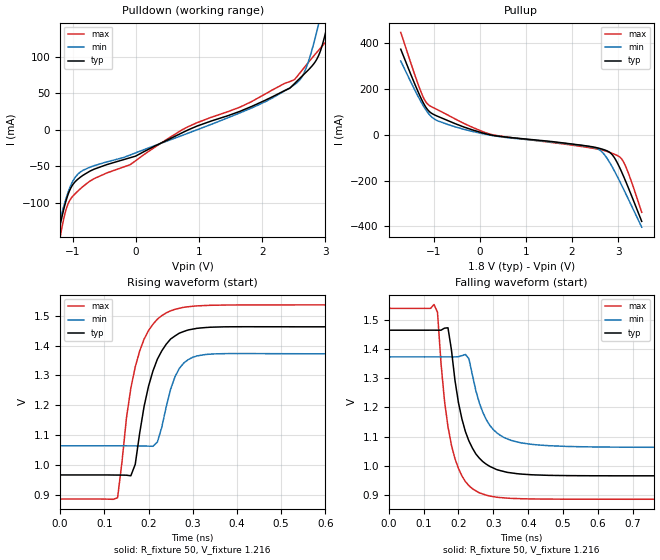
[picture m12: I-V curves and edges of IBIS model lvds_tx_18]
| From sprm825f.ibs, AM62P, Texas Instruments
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|   MODEL lvds_tx_18
[Model] lvds_tx_18
Model_type Output
C_comp 1.657p 1.754p 1.436p
Vmeas = 1.2
Vref = 1.2V
Rref = 50
Cref = 0.5pF
[Model Spec]
[Temperature Range]  40 150 -40
[Voltage Range] 1.8 1.62 1.98
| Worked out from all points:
|   slope of the pulldown table from 0 to 0.27 V, typ, clamps not added: 22.1 ohm
|   slope of the pullup table from 0 to 0.27 V, typ, clamps not added: 19.7 ohm
|   rising waveform, R_fixture 50, V_fixture 1.216: 20-80 % time 47.4ps typ, 35.3ps min, 46ps max; typ from 0.967 V to 1.46 V
|   falling waveform, R_fixture 50, V_fixture 1.216: 20-80 % time 54.9ps typ, 58.8ps min, 45.8ps max; typ from 1.46 V to 0.967 V
[Pulldown]
-1.71V    -377.9mA   -327mA     -450.5mA
-1.245V   -149.3mA   -138.7mA   -169.9mA
-1.193V   -127.2mA   -120.3mA   -143.1mA
-1.05V    -83.02mA   -79.84mA   -96.79mA
-838.9mV  -62.25mA   -55.44mA   -77.53mA
833.2mV   0A         -4.508mA   4.354mA
2.054V    40.45mA    38.4mA     49.03mA
2.624V    72.45mA    71.03mA    80.23mA
2.888V    99.94mA    141.8mA    107.9mA
3.03V     142mA      196.2mA    122.2mA
3.141V    189.6mA    241.3mA    140.8mA
3.511V    372.1mA    396.2mA    335.3mA
[Pullup]
-1.711V   372.1mA    320.5mA    445.6mA
-1.283V   163.7mA    147.3mA    191.7mA
-1.188V   126.6mA    114.7mA    149.3mA
-1.098V   102mA      89.24mA    128.1mA
-670.8mV  59.4mA     42.74mA    83.11mA
267.6mV   -2.529mA   -3.789mA   0A
2.565V    -58.29mA   -63.13mA   -63.53mA
2.702V    -66.38mA   -87.42mA   -69.87mA
2.855V    -84.19mA   -135.1mA   -80.46mA
3.088V    -168.2mA   -225.5mA   -109.5mA
3.235V    -239mA     -287.1mA   -175.4mA
3.51V     -377.9mA   -403.1mA   -338.5mA
[Ramp]
dV/dt_r .298/47.379p .185/34.618p .391/46.018p
dV/dt_f .298/54.889p .185/58.789p .391/45.304p
[Rising Waveform]
R_fixture = 50
V_fixture = 1.216
V_fixture_min = 1.219
V_fixture_max = 1.213
0s        967.5mV    1.065V     887.1mV
130ps     967.1mV    1.065V     891.3mV
160ps     964.8mV    1.065V     1.258V
170ps     1.003V     1.065V     1.329V
180ps     1.107V     1.065V     1.382V
200ps     1.264V     1.064V     1.45V
220ps     1.354V     1.077V     1.488V
250ps     1.422V     1.254V     1.516V
280ps     1.447V     1.342V     1.528V
3.73ns    1.463V     1.372V     1.537V
[Falling Waveform]
R_fixture = 50
V_fixture = 1.216
V_fixture_min = 1.219
V_fixture_max = 1.213
0s        1.464V     1.373V     1.538V
130ps     1.464V     1.373V     1.551V
140ps     1.464V     1.373V     1.525V
170ps     1.472V     1.373V     1.135V
190ps     1.293V     1.373V     1.026V
230ps     1.086V     1.367V     933.6mV
270ps     1.015V     1.183V     904.9mV
310ps     988.1mV    1.114V     894mV
600ps     967.1mV    1.065V     887.1mV
3.73ns    967.4mV    1.065V     886.8mV
